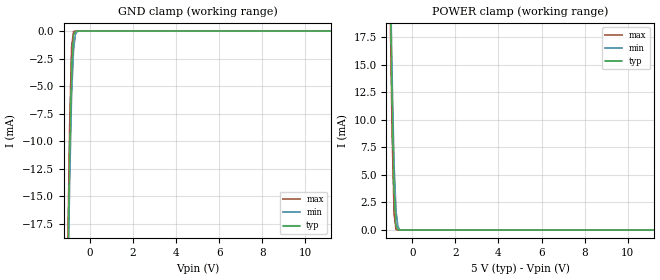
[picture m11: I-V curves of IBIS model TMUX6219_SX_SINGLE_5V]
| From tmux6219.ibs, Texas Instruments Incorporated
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[Model]   TMUX6219_SX_SINGLE_5V
Model_type   Terminator
|   typ   min   max
C_comp   32pF   32pF   32pF
[Voltage Range]   10   9   11
[Temperature Range]   27   125   -40
[Power Clamp Reference]   5   4.5   5.5
[GND Clamp Reference]   0   -0.5   -0.5
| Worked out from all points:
|   GND clamp passes 1 mA (typ) near -0.77 V on its own axis
|   POWER clamp passes 1 mA (typ) near -0.77 V on its own axis
[GND Clamp]
|   Voltage   I(typ)   I(min)   I(max)
-30V      -4.646A    -4.64A     -4.649A
-1.02V    -22.01mA   -24.41mA   -19.81mA
-930mV    -11.04mA   -13.89mA   -8.565mA
-840mV    -3.269mA   -5.934mA   -1.414mA
-750mV    -384.6uA   -1.761mA   -36.1uA
-660mV    -13.98uA   -270.8uA   -466nA
-570mV    -396.3nA   -19.97uA   -233nA
-210mV    0A         0A         0A
60V       0A         0A         0A
[POWER Clamp]
|   Voltage   I(typ)   I(min)   I(max)
-30V      4.646A     4.64A      4.649A
-1.02V    22.01mA    24.41mA    19.81mA
-930mV    11.04mA    13.89mA    8.565mA
-840mV    3.269mA    5.934mA    1.414mA
-750mV    384.6uA    1.761mA    36.1uA
-660mV    13.98uA    270.8uA    466nA
-570mV    396.3nA    19.97uA    233nA
-210mV    0A         0A         0A
60V       0A         0A         0A
